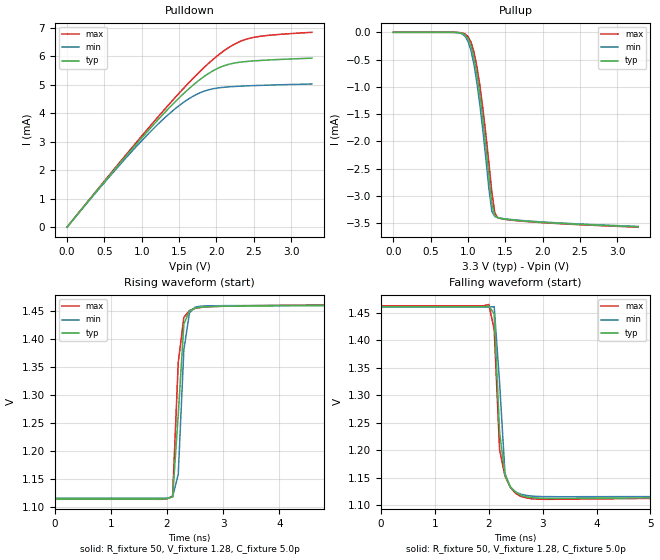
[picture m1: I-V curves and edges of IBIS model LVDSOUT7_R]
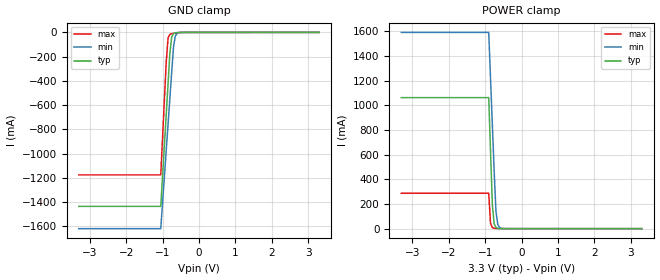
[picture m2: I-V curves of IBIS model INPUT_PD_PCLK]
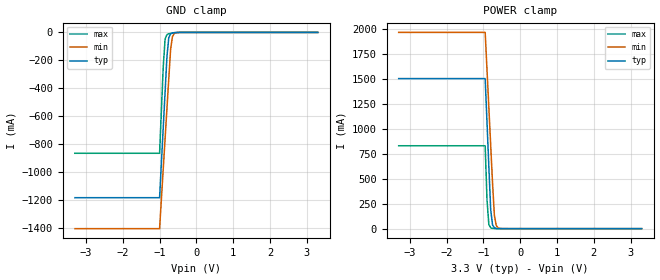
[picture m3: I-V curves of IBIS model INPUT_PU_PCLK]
|   This file is an IBIS representation of the   |
|   Integrated Device Technology, Inc.   |
|   ICS8543i   |
|   Low Skew 1 to 4 LVDS 3.3V Clock Buffer   |
[IBIS Ver]   4.0
[File name]   8543i_3v3.ibs
[File Rev]   1.0
[Date]   Aug 7  2007 | Last modified
|   Aug 7  2007 | Generated
[Source] Originated at Integrated Device Technology, Inc.
[Disclaimer]
IDT hereby grants the user of this IBIS model a non-exclusive,
nontransferable license to use this IBIS model under the following terms.
Before using this IBIS model, the user should read this license.
If the user does not accept these terms,  the IBIS model should be
returned to IDT within 30 days.
   The user is granted this license only to use the IBIS model and
is not granted rights to sell, load, rent, lease or license the IBIS
model in whole or in part, or in modified form to anyone other than
user. User may modify the IBIS model to suit its specific
applications but rights to derivative works and such modifications
shall belong to IDT.
   This IBIS model is provided on an "AS IS" basis and IDT makes
absolutely no warranty with respect to the information contained
herein. IDT DISCLAIMS AND CUSTOMER WAIVES ALL WARRANTIES, EXPRESS
OR IMPLIED, INCLUDING WARRANTIES OF MERCHANTABILITY OR FITNESS FOR
A PARTICULAR PURPOSE. The entire risk as to quality and performance
is with the Customer. ACCORDINGLY, IN NO EVENT SHALL THE COMPANY BE
LIABLE FOR ANY DAMAGES, WHETHER IN CONTRACT OR TORT,INCLUDING ANY
LOST PROFITS OR OTHER INCIDENTAL, CONSEQUENTIAL, EXEMPLARY, OR
PUNITIVE DAMAGES ARISING OUT OF THE USE OR APPLICATION OF THE IBIS
model provided in this package. Further, IDT reserves the right to
make changes without notice to any product herein to improve
reliability, function, or design. IDT does not convey any license
under patent rights or any other intellectual property rights,
including those of third parties.
   IDT is not obligated to provide maintenance or support
for the licensed IBIS model.
[Copyright]   Copyright 2007 by Integrated Device Technology, Inc.
[Component]   ICS8543BGI
[Manufacturer] Integrated Device Technology, Inc.
[Package]
|TSSOP 20 Lead
|   typ   min   max
R_pkg   51.85m   41.1m   62.6m
L_pkg   1.568nH   0.734nH   2.401nH
C_pkg   0.221pF   0.068pF   0.373pF
[Pin] signal_name  model_name   R_pin   L_pin   C_pin
1   GND   GND   62.6m   2.401n   0.373p
2   nRESET   INESD02_PU   57.23m   1.985n   0.297p
3   CLK_SEL   INESD02_PD   51.85m   1.568n   0.221p
4   CLK   INPUT_PD_CLK   46.78m   1.151n   0.145p
5   nCLK   INPUT_PU_CLK   41.1m   0.734n   0.068p
6   PCLK   INPUT_PD_PCLK  41.1m   0.734n   0.068p
7   nPCLK   INPUT_PU_PCLK  46.78m   1.151n   0.145p
8   OE   INESD02_PU   51.85m   1.568n   0.221p
9   GND   GND   57.23m   1.985n   0.297p
10   VDD   Power   62.6m   2.401n   0.373p
11   nQ3   LVDSOUT7_R   62.6m   2.401n   0.373p
12   Q3   LVDSOUT7_R   57.23m   1.985n   0.297p
13   GND   GND   51.85m   1.568n   0.221p
14   nQ2   LVDSOUT7_R   46.78m   1.151n   0.145p
15   Q2   LVDSOUT7_R   41.1m   0.734n   0.068p
16   nQ1   LVDSOUT7_R   41.1m   0.734n   0.068p
17   Q1   LVDSOUT7_R   46.78m   1.151n   0.145p
18   VDD   Power   51.85m   1.568n   0.221p
19   nQ0   LVDSOUT7_R   57.23m   1.985n   0.297p
20   Q0   LVDSOUT7_R   62.6m   2.401n   0.373p
[Diff Pin]  inv_pin  vdiff tdelay_typ tdelay_min  tdelay_max
|Output
12   11   0   0  0  0
15   14   0   0  0  0
17   16   0   0  0  0
20   19   0   0  0  0
|Input
4   5   0   0  0  0
6   7   0   0  0  0
| Models and submodels in the file (7): LVDSOUT7_R (Output), INPUT_PD_PCLK (Input_ECL), INPUT_PU_PCLK (Input_ECL), INPUT_PD_CLK (Input), INPUT_PU_CLK (Input), INESD02_PU (Input), INESD02_PD (Input)
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[Model]   LVDSOUT7_R
Model_type   Output
Polarity   Non-Inverting
Vmeas = 1.28
Rref = 50
Cref = 0
Vref = 1.28
|   typ   min   max
C_comp   2pF   1.5pF   2.5pF
|   typ   min   max
[Voltage range]  3.3V   3.15V   3.45V
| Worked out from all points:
|   slope of the pulldown table from 0 to 0.495 V, typ, clamps not added: 314 ohm
|   rising waveform, R_fixture 50, V_fixture 1.28, C_fixture 5.0p: 20-80 % time 133ps typ, 104ps min, 115ps max; typ from 1.11 V to 1.46 V
|   falling waveform, R_fixture 50, V_fixture 1.28, C_fixture 5.0p: 20-80 % time 137ps typ, 134ps min, 125ps max; typ from 1.46 V to 1.11 V
[pulldown]
|Voltage   I (typ)   I (min)   I (max)
0V        -48.44pA   -6.954pA   -1.112nA
600mV     1.906mA    1.864mA    1.935mA
1.04V     3.249mA    3.14mA     3.32mA
1.4V      4.27mA     4.049mA    4.407mA
1.56V     4.682mA    4.378mA    4.867mA
1.68V     4.965mA    4.58mA     5.197mA
1.84V     5.293mA    4.774mA    5.611mA
2.04V     5.597mA    4.89mA     6.065mA
2.2V      5.735mA    4.928mA    6.356mA
2.36V     5.8mA      4.951mA    6.559mA
2.64V     5.856mA    4.979mA    6.712mA
3.28V     5.929mA    5.023mA    6.835mA
[pullup]
|Voltage   I (typ)   I (min)   I (max)
0V        177.6pA    166.2pA    190.5pA
840mV     -1.878uA   -3.288uA   -1.043uA
1V        -112.8uA   -161.8uA   -77.15uA
1.08V     -463.4uA   -586.3uA   -359.2uA
1.16V     -1.15mA    -1.337mA   -980uA
1.24V     -2.09mA    -2.319mA   -1.873mA
1.28V     -2.62mA    -2.859mA   -2.39mA
1.32V     -3.144mA   -3.281mA   -2.928mA
1.36V     -3.363mA   -3.378mA   -3.314mA
1.4V      -3.398mA   -3.397mA   -3.397mA
1.64V     -3.445mA   -3.439mA   -3.451mA
3.28V     -3.564mA   -3.557mA   -3.57mA
[Ramp]
|   typ   min   max
dV/dt_r   0.24/0.3n   0.24/0.35n   0.24/0.25n
dV/dt_f   0.24/0.3n   0.24/0.35n   0.24/0.25n
[Rising Waveform]
R_fixture = 50
V_fixture = 1.28
V_fixture_max = 1.29
V_fixture_min = 1.27
C_fixture = 5.0p
| Time   typ   min   max
0s        1.114V     1.116V     1.114V
1.9ns     1.114V     1.116V     1.114V
2ns       1.115V     1.116V     1.115V
2.1ns     1.118V     1.118V     1.119V
2.2ns     1.265V     1.158V     1.358V
2.3ns     1.427V     1.381V     1.439V
2.4ns     1.451V     1.447V     1.451V
2.5ns     1.455V     1.457V     1.455V
3.2ns     1.459V     1.46V      1.459V
7ns       1.46V      1.46V      1.462V
[Falling Waveform]
R_fixture = 50
V_fixture = 1.28
V_fixture_max = 1.29
V_fixture_min = 1.27
C_fixture = 5.0p
| Time   typ   min   max
0s        1.461V     1.46V      1.462V
2ns       1.462V     1.46V      1.465V
2.1ns     1.448V     1.461V     1.42V
2.2ns     1.233V     1.323V     1.201V
2.3ns     1.155V     1.159V     1.153V
2.4ns     1.134V     1.133V     1.133V
2.5ns     1.123V     1.124V     1.121V
2.6ns     1.118V     1.12V      1.116V
3.1ns     1.112V     1.116V     1.111V
7ns       1.114V     1.116V     1.113V
[Model]   INPUT_PD_PCLK
Model_type   Input_ECL
Polarity   Non-Inverting
Vinl = 1.825V
Vinh = 2.135V
|   typ   min   max
C_comp   2pF   1.5pF   2.5pF
|   typ   min   max
[Voltage range]  3.3V   3.15V   3.45V
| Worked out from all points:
|   GND clamp passes 1 mA (typ) near -0.56 V on its own axis
|   POWER clamp passes 1 mA (typ) near -0.61 V on its own axis
[GND_clamp]
|Voltage   I(typ)   I(min)   I(max)
-3.3V     -1.436A    -1.62A     -1.176A
-1.05V    -1.436A    -1.62A     -1.176A
-900mV    -678.5mA   -975.1mA   -244mA
-850mV    -426.1mA   -760.1mA   -46.85mA
-800mV    -173.9mA   -545.4mA   -16.11mA
-750mV    -36.96mA   -330.7mA   -9.916mA
-700mV    -9.696mA   -120.2mA   -7.056mA
-650mV    -3.545mA   -29.7mA    -4.857mA
-600mV    -1.629mA   -7.52mA    -3.049mA
-400mV    -52.81uA   -52.52uA   -108.7uA
3.3V      71.13uA    77.43uA    62.11uA
[POWER_clamp]
|Voltage   I(typ)   I(min)   I(max)
-3.3V     1.063A     1.593A     287.3mA
-900mV    1.063A     1.593A     287.3mA
-850mV    620.5mA    1.215A     41.84mA
-800mV    191.6mA    837.5mA    8.757mA
-750mV    37.76mA    460.2mA    3.328mA
-700mV    8.104mA    133.8mA    1.728mA
-650mV    2.076mA    32.66mA    905.3uA
-600mV    678.1uA    8.083mA    443.8uA
-450mV    104.2uA    213.3uA    89.09uA
3.3V      -3.041nA   -3.986uA   0A
[Model]   INPUT_PU_PCLK
Model_type   Input_ECL
Polarity   Non-Inverting
Vinl = 1.825V
Vinh = 2.135V
|   typ   min   max
C_comp   2pF   1.5pF   2.5pF
|   typ   min   max
[Voltage range]  3.3V   3.15V   3.45V
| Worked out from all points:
|   GND clamp passes 1 mA (typ) near -0.56 V on its own axis
|   POWER clamp passes 1 mA (typ) near -0.61 V on its own axis
[GND_clamp]
|Voltage   I(typ)   I(min)   I(max)
-3.3V     -1.184A    -1.405A    -865.6mA
-1V       -1.184A    -1.405A    -865.6mA
-900mV    -678.5mA   -975.1mA   -244.1mA
-850mV    -426.2mA   -760.2mA   -46.92mA
-800mV    -174mA     -545.4mA   -16.17mA
-750mV    -37.03mA   -330.8mA   -9.981mA
-700mV    -9.767mA   -120.3mA   -7.122mA
-650mV    -3.616mA   -29.78mA   -4.922mA
-600mV    -1.7mA     -7.594mA   -3.115mA
-400mV    -123.9uA   -126uA     -173.9uA
3.3V      1.866nA    3.949uA    0A
[POWER_clamp]
|Voltage   I(typ)   I(min)   I(max)
-3.3V     1.506A     1.97A      832.1mA
-950mV    1.506A     1.97A      832.1mA
-900mV    1.063A     1.592A     287.2mA
-850mV    620.4mA    1.215A     41.77mA
-800mV    191.5mA    837.4mA    8.692mA
-750mV    37.69mA    460.1mA    3.262mA
-700mV    8.032mA    133.8mA    1.662mA
-650mV    2.005mA    32.58mA    840.1uA
-600mV    607uA      8.009mA    378.6uA
-450mV    33.11uA    139.8uA    23.88uA
3.3V      -71.13uA   -77.46uA   -62.11uA
